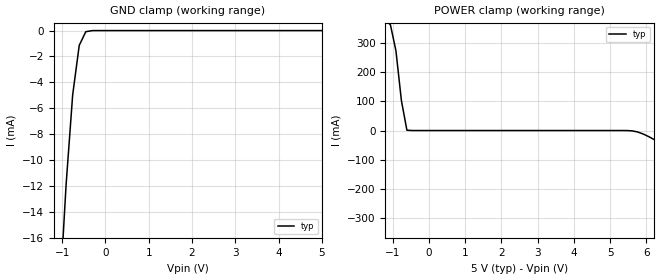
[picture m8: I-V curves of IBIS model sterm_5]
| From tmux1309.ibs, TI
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| sterm_5
[Model]   sterm_5
Model_type   Terminator
|   typ   min   max
C_comp   1.598234e-12   NA   NA
[Voltage Range]   5   NA   NA
[Temperature Range]   27   NA   NA
[Power Clamp Reference]   5   NA   NA
[GND Clamp Reference]   0   NA   NA
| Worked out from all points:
|   GND clamp passes 1 mA (typ) near -0.59 V on its own axis
|   POWER clamp passes 1 mA (typ) near -0.60 V on its own axis
[GND Clamp]
|   Voltage   I(typ)   I(min)   I(max)
-10V      -75.72kA   NA         NA
-1.061V   -20.75mA   NA         NA
-909.1mV  -11.88mA   NA         NA
-757.6mV  -4.963mA   NA         NA
-606.1mV  -1.14mA    NA         NA
-454.5mV  -87.23uA   NA         NA
-303mV    -1.844uA   NA         NA
5V        1.306nA    NA         NA
[POWER Clamp]
|   Voltage   I(typ)   I(min)   I(max)
-5V       1.511A     NA         NA
-1.061V   360.5mA    NA         NA
-909.1mV  272.4mA    NA         NA
-757.6mV  102mA      NA         NA
-606.1mV  1.019mA    NA         NA
5.455V    -87.23uA   NA         NA
5.758V    -4.963mA   NA         NA
6.061V    -20.75mA   NA         NA
6.515V    -53.61mA   NA         NA
7.879V    -171.4mA   NA         NA
8.03V     -404.4mA   NA         NA
10V       -20.06kA   NA         NA
